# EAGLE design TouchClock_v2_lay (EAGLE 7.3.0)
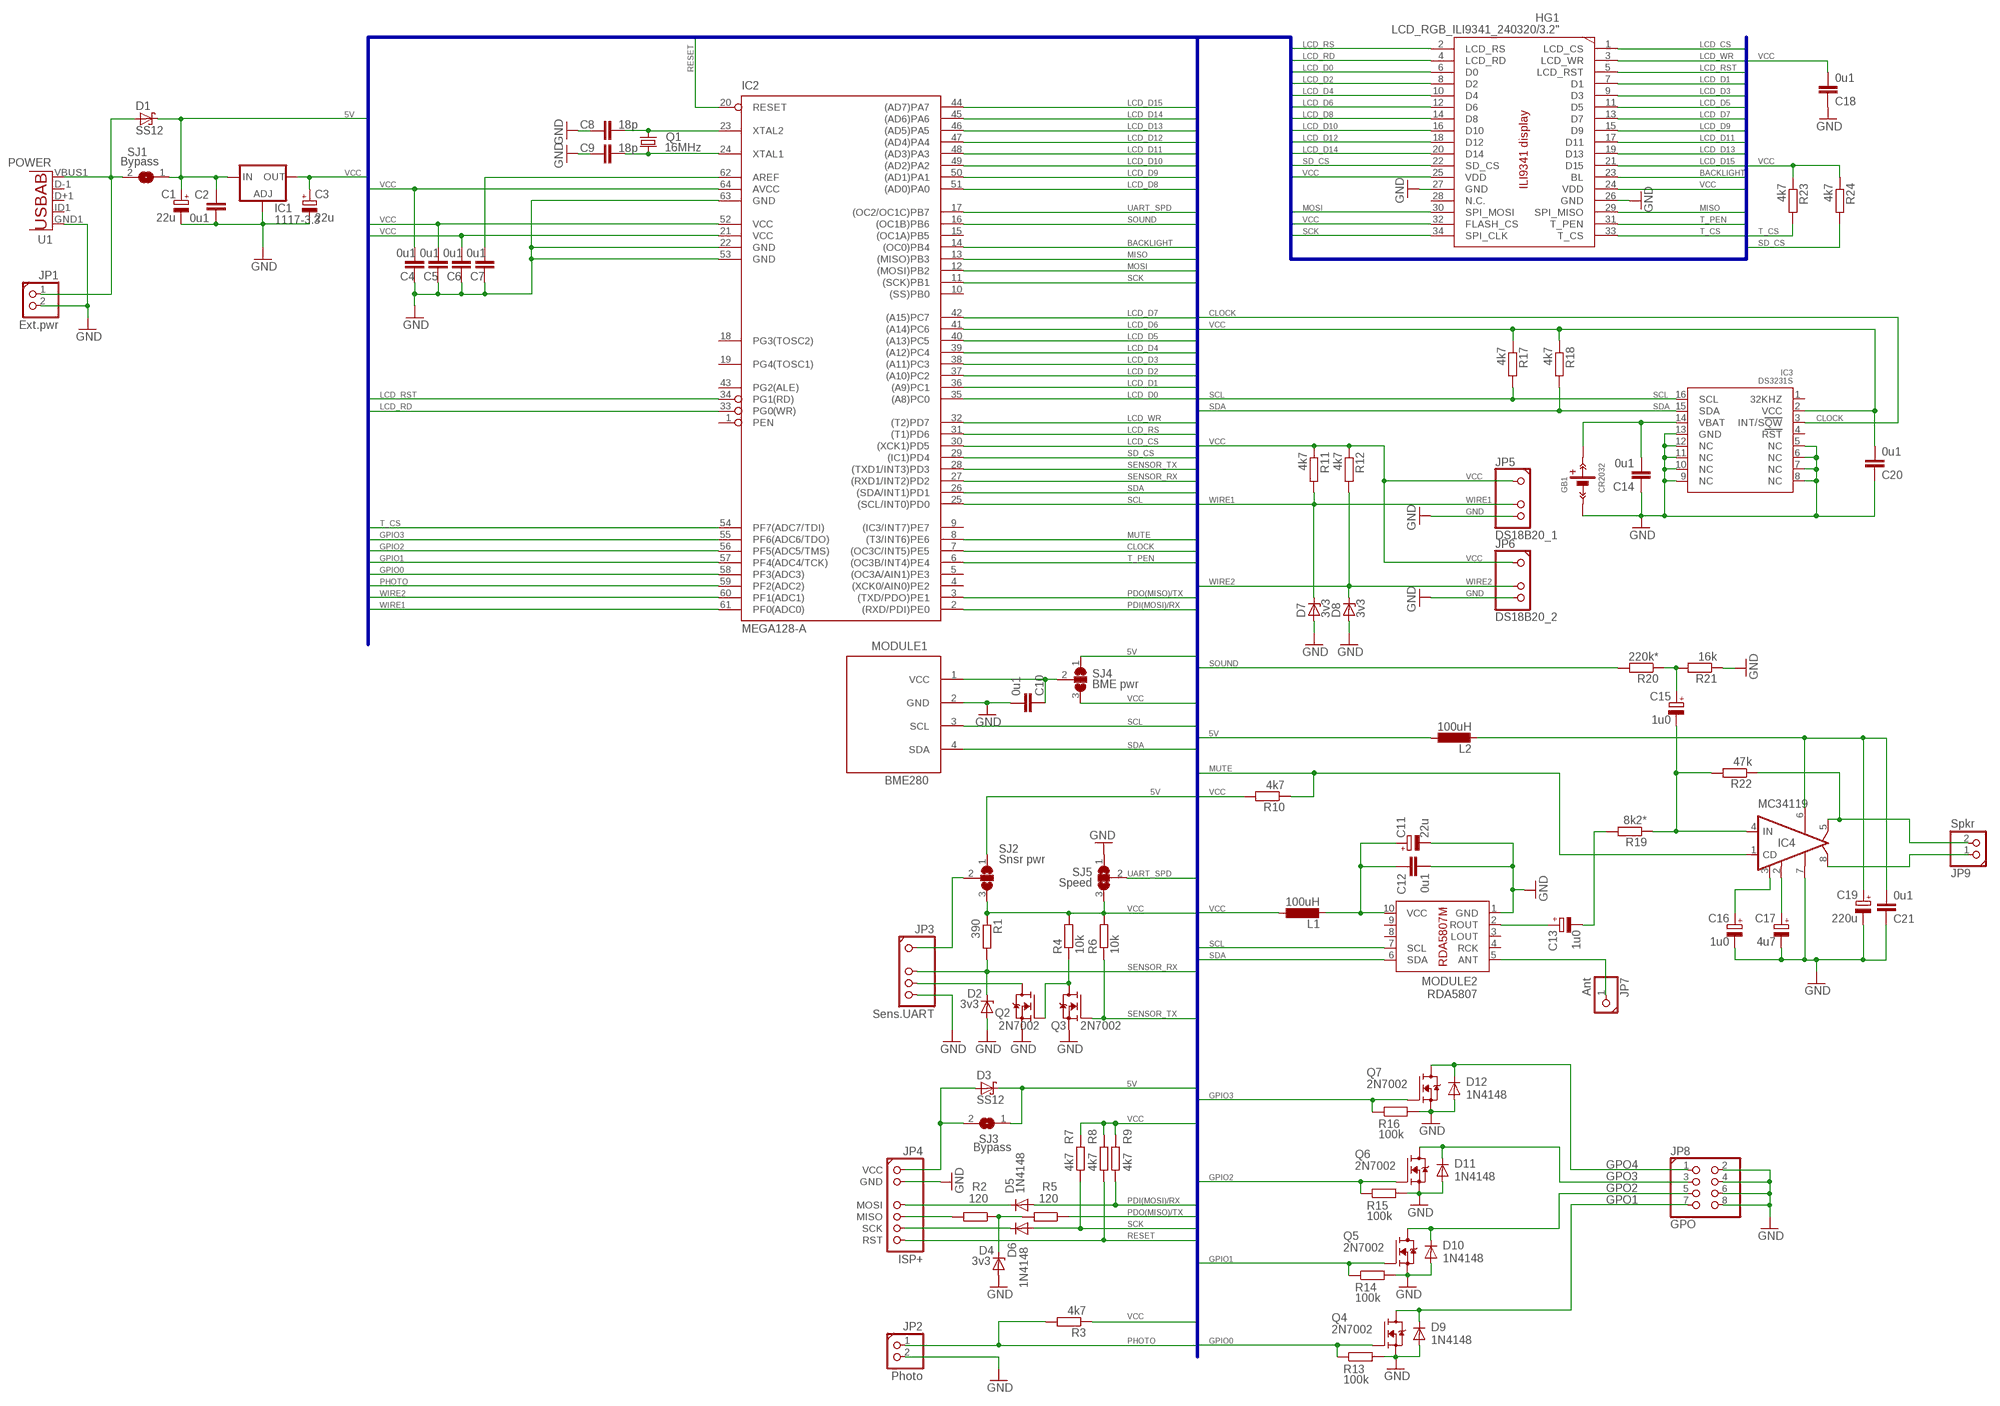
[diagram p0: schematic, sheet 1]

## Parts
C1  22u  CPOL-EUSMCB  [SMC_B]
C2  0u1  C-EUC0805T  [C0805T]
C3  22u  CPOL-EUSMCB  [SMC_B]
C4  0u1  C-EUC0805T  [C0805T]
C5  0u1  C-EUC0805T  [C0805T]
C6  0u1  C-EUC0805T  [C0805T]
C7  0u1  C-EUC0805T  [C0805T]
C8  18p  C-EUC0805T  [C0805T]
C9  18p  C-EUC0805T  [C0805T]
C10  0u1  C-EUC0805T  [C0805T]
C11  22u  CPOL-EUSMCB  [SMC_B]
C12  0u1  C-EUC0805T  [C0805T]
C13  1u0  CPOL-EUSMCB  [SMC_B]
C14  0u1  C-EUC0805T  [C0805T]
C15  1u0  CPOL-EUSMCB  [SMC_B]
C16  1u0  CPOL-EUSMCB  [SMC_B]
C17  4u7  CPOL-EUSMCB  [SMC_B]
C18  0u1  C-EUC0805T  [C0805T]
C19  220u  CPOL-EU153CLV-0605  [153CLV-0605]
C20  0u1  C-EUC0805T  [C0805T]
C21  0u1  C-EUC0805T  [C0805T]
D1  SS12  SS_XXX  [SMA(214AC)]
D2  3v3  ZENER-DIODESMB  [SMB(214AA)]
D3  SS12  SS_XXX  [SMA(214AC)]
D4  3v3  ZENER-DIODESOD80C  [SOD80C]
D5  1N4148  1N4148SMD  [SOD80-R]
D6  1N4148  1N4148SMD  [SOD80-R]
D7  3v3  ZENER-DIODESMB  [SMB(214AA)]
D8  3v3  ZENER-DIODESMB  [SMB(214AA)]
D9  1N4148  1N4148SMD  [SOD80-R]
D10  1N4148  1N4148SMD  [SOD80-R]
D11  1N4148  1N4148SMD  [SOD80-R]
D12  1N4148  1N4148SMD  [SOD80-R]
GB1  CR2032  CR2032_HOLDER/CH224  [CH224-2032]
HG1  LCD_RGB_ILI9341_240320/3.2"  [3"2_320*240_ILI9341]
IC1  1117-3.3  LD117AS33TR  [SOT223]
IC2  MEGA128-A  [TQFP64]
IC3  DS3231S  [SO16W]
IC4  MC34119  MC34119D  [SO08]
JP1  Ext.pwr  CONN1X2/R  [1X02ROUND]
JP2  Photo  CONN1X2/R  [1X02ROUND]
JP3  Sens.UART  CONN1X5(1+3)90R  [1X05ROUND/90(1+3)]
JP4  ISP+  CONN1X7(2+4)_ISP+/R90  [1X07/90/R_ISP+]
JP5  DS18B20_1  CONN1X4(1+2)/R90  [1X04ROUND/90(1+2)]
JP6  DS18B20_2  CONN1X4(1+2)/R90  [1X04ROUND/90(1+2)]
JP7  Ant  CONN1X1/R90  [1X01ROUND/90]
JP8  GPO  CONN2X4/R  [2X04ROUND]
JP9  Spkr  CONN1X2/R90  [1X02ROUND/90]
L1  100uH  L-EUL1812  [L1812]
L2  100uH  L-EUL1812  [L1812]
MODULE1  BME280  BM(P|E)280_I2C/4  [BM(P|E)280_I2C_5V]
MODULE2  RDA5807  RDA5807M/PAD  [RDA5807_MODULE_PADS]
Q1  16MHz  CRYSTALSM49  [SM49]
Q2  2N7002  2N7002/THIN  [SOT23_THIN]
Q3  2N7002  2N7002/THIN  [SOT23_THIN]
Q4  2N7002  2N7002/THIN  [SOT23_THIN]
Q5  2N7002  2N7002/THIN  [SOT23_THIN]
Q6  2N7002  2N7002/THIN  [SOT23_THIN]
Q7  2N7002  2N7002/THIN  [SOT23_THIN]
R1  390  R-EU_R0805T  [R0805T]
R2  120  R-EU_R0805T  [R0805T]
R3  4k7  R-EU_R0805T  [R0805T]
R4  10k  R-EU_R0805T  [R0805T]
R5  120  R-EU_R0805T  [R0805T]
R6  10k  R-EU_R0805T  [R0805T]
R7  4k7  R-EU_R0805T  [R0805T]
R8  4k7  R-EU_R0805T  [R0805T]
R9  4k7  R-EU_R0805T  [R0805T]
R10  4k7  R-EU_R0805T  [R0805T]
R11  4k7  R-EU_R0805T  [R0805T]
R12  4k7  R-EU_R0805T  [R0805T]
R13  100k  R-EU_R0805T  [R0805T]
R14  100k  R-EU_R0805T  [R0805T]
R15  100k  R-EU_R0805T  [R0805T]
R16  100k  R-EU_R0805T  [R0805T]
R17  4k7  R-EU_R0805T  [R0805T]
R18  4k7  R-EU_R0805T  [R0805T]
R19  8k2*  R-EU_R0805T  [R0805T]
R20  220k*  R-EU_R0805T  [R0805T]
R21  16k  R-EU_R0805T  [R0805T]
R22  47k  R-EU_R0805T  [R0805T]
R23  4k7  R-EU_R0805T  [R0805T]
R24  4k7  R-EU_R0805T  [R0805T]
SJ1  Bypass  SJ/NS  [SJ_NOSILK]
SJ2  Snsr pwr  SJ2W  [SJ_2]
SJ3  Bypass  SJ/NS  [SJ_NOSILK]
SJ4  BME pwr  SJ2W  [SJ_2]
SJ5  Speed  SJ2W  [SJ_2]
U1  POWER  USB5""  [USB-MICRO-SMD]

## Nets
5V: C1.+ C2.1 D1.C D3.C IC1.3(IN) L2.1 SJ1.1 SJ2.1 SJ3.1 SJ4.1
BACKLIGHT: HG1.23(BL) IC2.14((OC0)PB4)
CLOCK: IC2.7((OC3C/INT5)PE5) IC3.3(INT/SQW)
GND: C1.- C2.2 C3.- C4.1 C5.1 C6.1 C7.1 C8.1 C9.1 C10.2 C11.- C12.2 C14.1 C16.- C17.- C18.1 C19.- C20.1 C21.1 D2.A D4.A D7.A D8.A D9.A D10.A D11.A D12.A GB1.GB- HG1.26(GND) HG1.27(GND) IC1.1(ADJ) IC2.22(GND) IC2.53(GND) IC2.63(GND) IC3.5(NC) IC3.6(NC) IC3.7(NC) IC3.8(NC) IC3.9(NC) IC3.10(NC) IC3.11(NC) IC3.12(NC) IC3.13(GND) IC4.7(GND) JP1.2 JP2.2 JP3.5 JP4.GND JP5.4 JP6.4 JP8.2 JP8.4 JP8.6 JP8.8 MODULE1.2(GND) MODULE2.1(GND) Q2.2(S) Q3.2(S) Q4.2(S) Q5.2(S) Q6.2(S) Q7.2(S) R13.2 R14.2 R15.2 R16.2 R21.1 SJ5.1 U1.GND1(GND)
GPIO0: IC2.58(PF3(ADC3)) Q4.1(G) R13.1
GPIO1: IC2.57(PF4(ADC4/TCK)) Q5.1(G) R14.1
GPIO2: IC2.56(PF5(ADC5/TMS)) Q6.1(G) R15.1
GPIO3: IC2.55(PF6(ADC6/TDO)) Q7.1(G) R16.1
GPO1: D9.C JP8.7 Q4.3(D)
GPO2: D10.C JP8.5 Q5.3(D)
GPO3: D11.C JP8.3 Q6.3(D)
GPO4: D12.C JP8.1 Q7.3(D)
LCD_CS: HG1.1(LCD_CS) IC2.30((XCK1)PD5)
LCD_D0: HG1.6(D0) IC2.35((A8)PC0)
LCD_D1: HG1.7(D1) IC2.36((A9)PC1)
LCD_D2: HG1.8(D2) IC2.37((A10)PC2)
LCD_D3: HG1.9(D3) IC2.38((A11)PC3)
LCD_D4: HG1.10(D4) IC2.39((A12)PC4)
LCD_D5: HG1.11(D5) IC2.40((A13)PC5)
LCD_D6: HG1.12(D6) IC2.41((A14)PC6)
LCD_D7: HG1.13(D7) IC2.42((A15)PC7)
LCD_D8: HG1.14(D8) IC2.51((AD0)PA0)
LCD_D9: HG1.15(D9) IC2.50((AD1)PA1)
LCD_D10: HG1.16(D10) IC2.49((AD2)PA2)
LCD_D11: HG1.17(D11) IC2.48((AD3)PA3)
LCD_D12: HG1.18(D12) IC2.47((AD4)PA4)
LCD_D13: HG1.19(D13) IC2.46((AD5)PA5)
LCD_D14: HG1.20(D14) IC2.45((AD6)PA6)
LCD_D15: HG1.21(D15) IC2.44((AD7)PA7)
LCD_RD: HG1.4(LCD_RD) IC2.33(PG0(WR))
LCD_RS: HG1.2(LCD_RS) IC2.31((T1)PD6)
LCD_RST: HG1.5(LCD_RST) IC2.34(PG1(RD))
LCD_WR: HG1.3(LCD_WR) IC2.32((T2)PD7)
MISO: HG1.29(SPI_MISO) IC2.13((MISO)PB3)
MOSI: HG1.30(SPI_MOSI) IC2.12((MOSI)PB2)
MUTE: IC2.8((T3/INT6)PE6) IC4.1(CD) R10.1
N$1: C9.2 IC2.24(XTAL1) Q1.2
N$2: C8.2 IC2.23(XTAL2) Q1.1
N$3: C7.2 IC2.62(AREF)
N$4: JP4.MISO R2.2
N$5: C16.+ IC4.3(FC1)
N$6: C11.+ C12.1 L1.2 MODULE2.10(VCC)
N$7: C17.+ IC4.2(FC2)
N$8: JP7.1 MODULE2.5(ANT)
N$9: C13.+ MODULE2.2(ROUT)
N$10: C13.- R19.2
N$11: C19.+ C21.2 IC4.6(VCC) L2.2
N$12: C15.+ R20.1 R21.2
N$13: C15.- IC4.4(IN) R19.1 R22.2
N$14: IC4.8(VO2) JP9.1
N$15: IC4.5(VO1) JP9.2 R22.1
N$16: JP3.1 SJ2.2
N$17: JP3.4 Q2.3(D)
N$18: D4.C R2.1 R5.2
N$19: Q2.1(G) Q3.3(D) R4.1
N$20: C10.1 MODULE1.1(VCC) SJ4.2
N$23: D3.A JP4.+5V(VCC) SJ3.2
N$25: D5.C JP4.MOSI
N$26: D6.C JP4.SCK
PDI(MOSI)/RX: D5.A IC2.2((RXD/PDI)PE0) R9.2
PDO(MISO)/TX: IC2.3((TXD/PDO)PE1) R5.1
PHOTO: IC2.59(PF2(ADC2)) JP2.1 R3.2
RESET: IC2.20(RESET) JP4.RST R8.2
SCK: D6.A HG1.34(SPI_CLK) IC2.11((SCK)PB1) R7.2
SCL: IC2.25((SCL/INT0)PD0) IC3.16(SCL) MODULE1.3(SCL) MODULE2.7(SCL) R17.2
SD_CS: HG1.22(SD_CS) IC2.29((IC1)PD4) R24.2
SDA: IC2.26((SDA/INT1)PD1) IC3.15(SDA) MODULE1.4(SDA) MODULE2.6(SDA) R18.2
SENSOR_RX: D2.C IC2.27((RXD1/INT2)PD2) JP3.3 R1.2
SENSOR_TX: IC2.28((TXD1/INT3)PD3) Q3.1(G) R6.1
SOUND: IC2.16((OC1B)PB6) R20.2
SUPPLY: D1.A JP1.1 SJ1.2 U1.VBUS1(VBUS)
T_CS: HG1.33(T_CS) IC2.54(PF7(ADC7/TDI)) R23.2
T_PEN: HG1.31(T_PEN) IC2.6((OC3B/INT4)PE4)
UART_SPD: IC2.17((OC2/OC1C)PB7) SJ5.2
VBAT: C14.2 GB1.GB+ IC3.14(VBAT)
VCC: C3.+ C4.2 C5.2 C6.2 C18.2 C20.2 HG1.24(VDD) HG1.25(VDD) HG1.32(FLASH_CS) IC1.4(OUT) IC2.21(VCC) IC2.52(VCC) IC2.64(AVCC) IC3.2(VCC) JP5.1 JP6.1 L1.1 R1.1 R3.1 R4.2 R6.2 R7.1 R8.1 R9.1 R10.2 R11.1 R12.1 R17.1 R18.1 R23.1 R24.1 SJ2.3 SJ4.3 SJ5.3
WIRE1: D7.C IC2.61(PF0(ADC0)) JP5.3 R11.2
WIRE2: D8.C IC2.60(PF1(ADC1)) JP6.3 R12.2
Unconnected: HG1.28(N.C.) IC2.1(PEN) IC2.4((XCK0/AIN0)PE2) IC2.5((OC3A/AIN1)PE3) IC2.9((IC3/INT7)PE7) IC2.10((SS)PB0) IC2.15((OC1A)PB5) IC2.18(PG3(TOSC2)) IC2.19(PG4(TOSC1)) IC2.43(PG2(ALE)) IC3.1(32KHZ) IC3.4(RST) MODULE2.3(LOUT) MODULE2.4(RCK) MODULE2.8(NC1) MODULE2.9(NC2) U1.D+1(D+) U1.D-1(D-) U1.ID1(USBID)

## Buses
5V,VCC,LCD_CS,LCD_WR,LCD_RD,LCD_RST,LCD_RS,LCD_D[0..15],MISO,MOSI,SCK,PDI(MOSI)/RX,PDO(MISO)/TX,T_PEN,T_CS,SD_CS,BACKLIGHT,RESET,SCL,SDA,WIRE1,WIRE2,CLOCK,SOUND,MUTE,SENSOR_RX,SENSOR_TX,GPIO[0..3],PHOTO,UART_SPD

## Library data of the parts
C1 C3 C11 C13 C15-C17 C19 = rcl:CPOL-EU: POLARIZED CAPACITOR, European symbol
C2 C4-C10 C12 C14 C18 C20 C21 = rcl:C-EU: CAPACITOR, European symbol
D1 D3 = diode:SS_XXX: SS12 -13 -14 -15 -16 -18 -19 -100
D2 D4 D7 D8 = diode:ZENER-DIODE: Z-Diode
D5 D6 D9-D12 = diode:1N4148: DIODE
GB1 = misc_passive_AL:CR2032_HOLDER: CR2032 Holder
HG1 = lcd-AL:LCD_RGB_ILI9341_240*320
IC1 = v-reg:LD117A?*: Low drop fixed and adjustable positive voltage regulators 1 A Source: http://www.st.com/stonline/products/literature/ds/7194/ld1117axx.pdf
IC2 = atmel:MEGA128: MICROCONTROLLER 128 Kbytes FLASH 4 Kbytes SRAM 4 Kbytes EEPROM DUAL USART 8-channel 10 bit ADC Source: avr.lbr; MPN: ATMEGA128-16AU; OC_FARNELL: 9171118; OC_NEWARK: 95K7364
IC3 = misc-active-AL:DS3231S: TCXO Clock
IC4 = misc-active-AL:MC34119: Low Power Audio Amplifier Motorola
JP1 JP2 JP9 = pinhead-AL:CONN1X2: PIN HEADER
JP3 = pinhead-AL:CONN1X5(1+3)
JP4 = pinhead-AL:CONN1X7(2+4)_ISP+: PIN HEADER
JP5 JP6 = pinhead-AL:CONN1X4(1+2)
JP7 = pinhead-AL:CONN1X1
JP8 = pinhead-AL:CONN2X4: PIN HEADER
L1 L2 = rcl:L-EU: INDUCTOR, European symbol
MODULE1 = modules-external-AL:BM(P|E)280_I2C
MODULE2 = modules-external-AL:RDA5807M
Q1 = crystal:CRYSTAL: CRYSTAL; OC_FARNELL: unknown; OC_NEWARK: unknown
Q2-Q7 = transistor-fet:2N7002: Small signal N-Channel MOSFET transistor
R1-R24 = rcl:R-EU_: RESISTOR, European symbol
SJ1 SJ3 = jumper:SJ: SMD solder JUMPER
SJ2 SJ4 SJ5 = jumper:SJ2W: SMD solder JUMPER
U1 = usb:USB5: This is a USB AB connector that is compatible with USB OTG. i.e. this connector can serve as a host or device

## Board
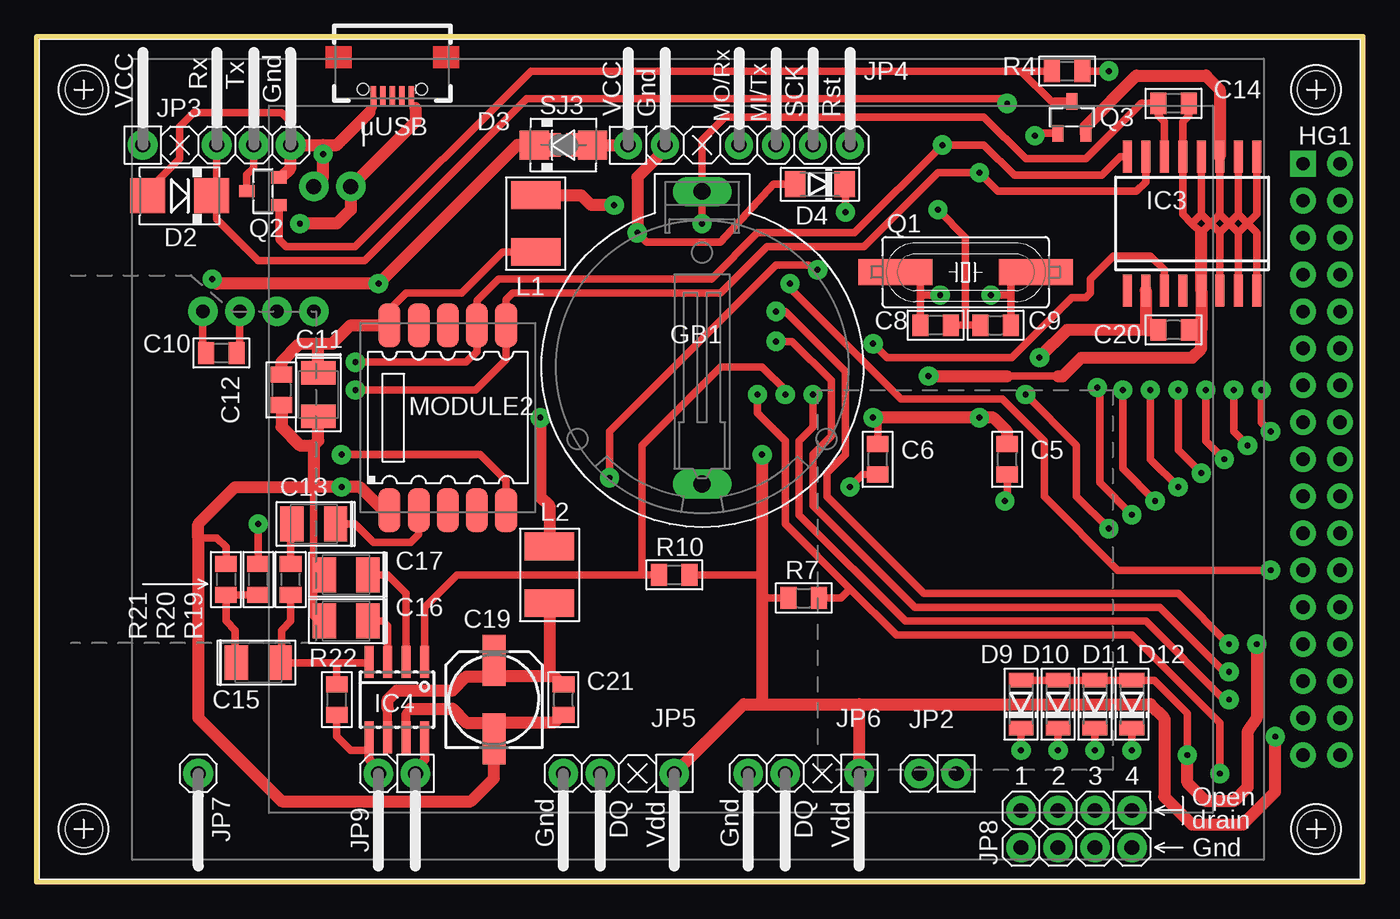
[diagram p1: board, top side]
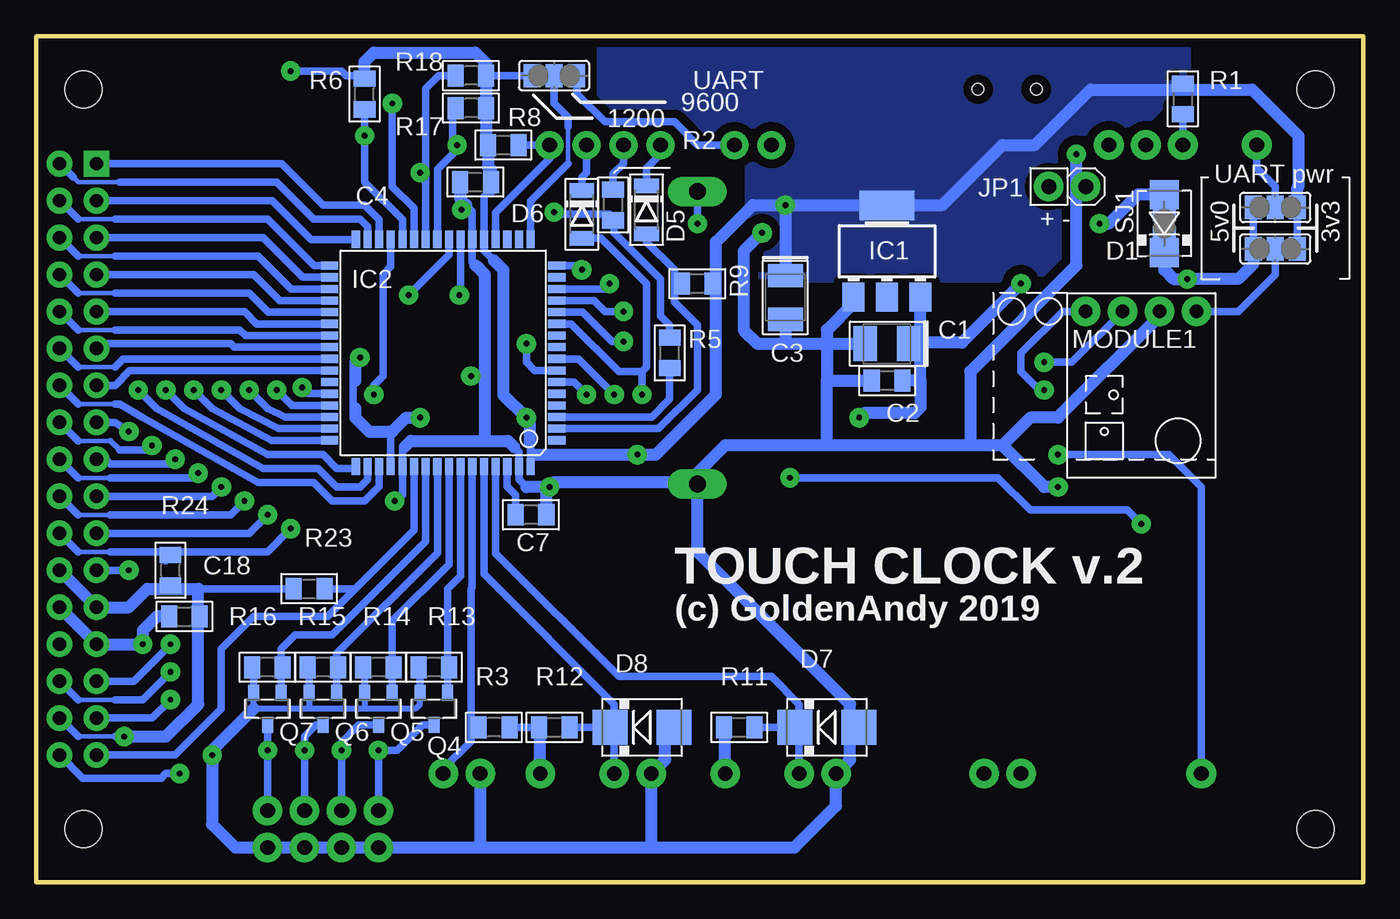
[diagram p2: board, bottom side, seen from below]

Size 91.12 x 58.1 mm. Coordinates in mm from the lower left corner, seen from the top.
Outline: 0,58.1 91.12,58.1 91.12,0 0,0 0,58.1
Copper layers (1*16): Top 0.035mm / dielectric 1.5mm / Bottom 0.035mm
Design rules "default *": minimum track width 12mil, minimum drill 14mil, track to track 8mil, track to pad 8mil, pad to pad 8mil, via to via 8mil, smd to smd 8mil, copper to edge 20mil, drill to drill 30mil, minimum pad ring 16mil, minimum via ring 18mil, stop-mask expansion 4mil, vias tented up to drill 0mil, thermal gap 16mil
Holes 2.54 mm at 3.25,54.45 87.89,54.45 87.89,3.65 3.25,3.65

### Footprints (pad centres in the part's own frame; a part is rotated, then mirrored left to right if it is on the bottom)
SMC_B = smd 1.6 x 2.4: + -1.5,0; - 1.5,0
C0805T = smd 1.1 x 1.5: 1 -1.05,0; 2 1.05,0
153CLV-0605 = smd 3.5 x 1.6: + 2.7,0; - -2.7,0
SMA(214AC) = smd 2 x 2: A 2,0; C -2,0
SMB(214AA) = smd 2.4 x 2.4: A 2.2,0; C -2.2,0
SOD80C = smd 1.4 x 1.8: A 1.7,0; C -1.7,0
SOD80-R = smd 1 x 1.7: A 1.65,0; C -1.65,0
CH224-2032 = drill 1.143 pad 2.032 long: GB+ -12.05,0; GB- 8.05,0
3"2_320*240_ILI9341 = drill 0.9 pad 1.778 square: 1 32.703,20.32 | drill 0.9 pad 1.778: 2 35.242,20.32; 3 32.703,17.78; 4 35.242,17.78; 5 32.703,15.24; 6 35.242,15.24; 7 32.703,12.7; 8 35.242,12.7; 9 32.703,10.16; 10 35.242,10.16; 11 32.703,7.62; 12 35.242,7.62; 13 32.703,5.08; 14 35.242,5.08; 15 32.703,2.54; 16 35.242,2.54; 17 32.703,0; 18 35.242,0; 19 32.703,-2.54; 20 35.242,-2.54; 21 32.703,-5.08; 22 35.242,-5.08; 23 32.703,-7.62; 24 35.242,-7.62; 25 32.703,-10.16; 26 35.242,-10.16; 27 32.703,-12.7; 28 35.242,-12.7; 29 32.703,-15.24; 30 35.242,-15.24; 31 32.703,-17.78; 32 35.242,-17.78; 33 32.703,-20.32; 34 35.242,-20.32
SOT223 = smd 1.5 x 2: 1 -2.3,-3.15; 2 0,-3.15; 3 2.3,-3.15 | smd 3.8 x 2: 4 0,3.15
TQFP64 = smd 1.194 x 0.559: 1 -7.8,6; 2 -7.8,5.2; 3 -7.8,4.4; 4 -7.8,3.6; 5 -7.8,2.8; 6 -7.8,2; 7 -7.8,1.2; 8 -7.8,0.4; 9 -7.8,-0.4; 10 -7.8,-1.2; 11 -7.8,-2; 12 -7.8,-2.8; 13 -7.8,-3.6; 14 -7.8,-4.4; 15 -7.8,-5.2; 16 -7.8,-6; 33 7.8,-6; 34 7.8,-5.2; 35 7.8,-4.4; 36 7.8,-3.6; 37 7.8,-2.8; 38 7.8,-2; 39 7.8,-1.2; 40 7.8,-0.4; 41 7.8,0.4; 42 7.8,1.2; 43 7.8,2; 44 7.8,2.8; 45 7.8,3.6; 46 7.8,4.4; 47 7.8,5.2; 48 7.8,6 | smd 0.559 x 1.194: 17 -6,-7.8; 18 -5.2,-7.8; 19 -4.4,-7.8; 20 -3.6,-7.8; 21 -2.8,-7.8; 22 -2,-7.8; 23 -1.2,-7.8; 24 -0.4,-7.8; 25 0.4,-7.8; 26 1.2,-7.8; 27 2,-7.8; 28 2.8,-7.8; 29 3.6,-7.8; 30 4.4,-7.8; 31 5.2,-7.8; 32 6,-7.8; 49 6,7.8; 50 5.2,7.8; 51 4.4,7.8; 52 3.6,7.8; 53 2.8,7.8; 54 2,7.8; 55 1.2,7.8; 56 0.4,7.8; 57 -0.4,7.8; 58 -1.2,7.8; 59 -2,7.8; 60 -2.8,7.8; 61 -3.6,7.8; 62 -4.4,7.8; 63 -5.2,7.8; 64 -6,7.8
SO16W = smd 0.6 x 2.2: 1 -4.445,-4.6; 2 -3.175,-4.6; 3 -1.905,-4.6; 4 -0.635,-4.6; 5 0.635,-4.6; 6 1.905,-4.6; 7 3.175,-4.6; 8 4.445,-4.6; 9 4.445,4.6; 10 3.175,4.6; 11 1.905,4.6; 12 0.635,4.6; 13 -0.635,4.6; 14 -1.905,4.6; 15 -3.175,4.6; 16 -4.445,4.6
SO08 = smd 0.6 x 2.2: 1 -1.905,-2.6; 2 -0.635,-2.6; 3 0.635,-2.6; 4 1.905,-2.6; 5 1.905,2.6; 6 0.635,2.6; 7 -0.635,2.6; 8 -1.905,2.6
1X02ROUND = drill 1.016 pad 2.032: 1 -1.27,0; 2 1.27,0
1X05ROUND/90(1+3) = drill 1.016 pad 2.032: 1 -5.08,0; 3 0,0; 4 2.54,0; 5 5.08,0
1X07/90/R_ISP+ = drill 1.016 pad 1.93: +5V -7.62,0; GND -5.08,0; MISO 2.54,0; MOSI 0,0; RST 7.62,0; SCK 5.08,0
1X04ROUND/90(1+2) = drill 1.016 pad 2.032: 1 -3.81,0; 3 1.27,0; 4 3.81,0
1X01ROUND/90 = drill 1.016 pad 2.032: 1 0,0
2X04ROUND = drill 1.016 pad 2.032: 1 -3.81,-1.27; 2 -3.81,1.27; 3 -1.27,-1.27; 4 -1.27,1.27; 5 1.27,-1.27; 6 1.27,1.27; 7 3.81,-1.27; 8 3.81,1.27
1X02ROUND/90 = drill 1.016 pad 2.032: 1 -1.27,0; 2 1.27,0
L1812 = smd 1.9 x 3.4: 1 -1.95,0; 2 1.95,0
BM(P|E)280_I2C_5V = drill 0.914 pad 2.032: 1 3.81,5.08; 2 1.27,5.08; 3 -1.27,5.08; 4 -3.81,5.08
RDA5807_MODULE_PADS = smd 3.048 x 1.524: 1 -6.35,4; 2 -6.35,2; 3 -6.35,0; 4 -6.35,-2; 5 -6.35,-4; 6 6.35,-4; 7 6.35,-2; 8 6.35,0; 9 6.35,2; 10 6.35,4
SM49 = smd 5.08 x 1.778: 1 -4.826,0; 2 4.826,0
SOT23_THIN = smd 0.8 x 1.1: 1 -0.95,-1.1; 2 0.95,-1.1; 3 0,1.1
R0805T = smd 1.1 x 1.5: 1 -1.05,0; 2 1.05,0
SJ_NOSILK = smd 1.168 x 1.6: 1 -0.762,0; 2 0.762,0
SJ_2 = smd 1.168 x 1.6: 1 -1.524,0; 2 0,0; 3 1.524,0
USB-MICRO-SMD = smd 1.4 x 0.4: D+1 2.7,0; D-1 2.7,0.65; GND1 2.7,-1.3; ID1 2.7,-0.65; VBUS1 2.7,1.3 | hole 0.8: 2.2,2; 2.2,-2

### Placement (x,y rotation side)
C1  32.7,36.99 180 bottom
C2  32.7,34.45 180 bottom
C3  39.69,40.16 270 bottom
C4  60.96,48.1 0 bottom
C5  66.67,29.05 90 top
C6  57.79,29.05 90 top
C7  57.15,25.24 180 bottom
C8  61.75,38.26 180 top
C9  65.88,38.26 0 top
C10  12.7,36.35 0 top
C11  19.37,33.5 270 top
C12  16.83,33.81 270 top
C13  19.05,24.61 180 top
C14  78.11,53.5 180 top
C15  15.24,15.08 0 top
C16  21.27,17.94 180 top
C17  21.27,21.11 180 top
C18  80.96,18.26 0 bottom
C19  31.43,12.54 90 top
C20  78.11,37.94 180 top
C21  36.2,12.54 90 top
D1  13.65,45.24 90 bottom
D2  9.84,47.15 180 top
D3  36.2,50.64 0 top
D4  53.82,47.94 180 top
D5  49.21,46.2 270 bottom
D6  53.66,45.88 270 bottom
D7  36.83,10.64 0 bottom
D8  49.53,10.64 0 bottom
D9  67.63,12.22 90 top
D10  70.17,12.22 90 top
D11  72.71,12.22 90 top
D12  75.25,12.22 90 top
GB1  45.72,35.4 270 top
HG1  54.29,29.05 0 top
IC1  32.7,43.34 0 bottom
IC2  63.18,36.35 180 bottom
IC3  79.38,45.24 0 top
IC4  24.77,12.54 180 top
JP1  20.32,47.78 0 bottom
JP2  61.91,7.46 180 top
JP3  12.38,50.64 0 top
JP4  48.26,50.64 0 top
JP5  40.01,7.46 180 top
JP6  52.71,7.46 180 top
JP7  11.11,7.46 180 top
JP8  71.44,3.65 180 top
JP9  24.77,7.46 180 top
L1  34.29,45.24 270 top
L2  35.24,21.11 270 top
MODULE1  15.24,34.13 0 bottom
MODULE2  28.26,31.91 90 top
Q1  63.82,41.91 0 top
Q2  15.56,47.47 90 top
Q3  71.12,52.55 0 top
Q4  63.82,11.91 180 bottom
Q5  67.63,11.91 180 bottom
Q6  71.44,11.91 180 bottom
Q7  75.25,11.91 180 bottom
R1  12.38,53.82 270 bottom
R2  51.51,46.51 90 bottom
R3  59.69,10.64 180 bottom
R4  70.8,55.72 0 top
R5  47.62,36.35 90 bottom
R6  68.58,54.13 90 bottom
R7  52.71,19.53 0 top
R8  59.05,50.64 0 bottom
R9  45.72,41.12 180 bottom
R10  43.82,21.11 0 top
R11  42.86,10.64 0 bottom
R12  55.56,10.64 0 bottom
R13  63.82,14.76 180 bottom
R14  67.63,14.76 180 bottom
R15  71.44,14.76 180 bottom
R16  75.25,14.76 180 bottom
R17  61.28,53.18 180 bottom
R18  61.28,55.4 180 bottom
R19  17.46,20.8 90 top
R20  15.24,20.8 90 top
R21  13.02,20.8 270 top
R22  20.64,12.54 90 top
R23  72.39,20.16 0 bottom
R24  81.92,21.43 90 bottom
SJ1  13.65,45.24 90 bottom
SJ2  6.03,46.36 0 bottom
SJ3  36.2,50.64 0 top
SJ4  6.03,43.5 0 bottom
SJ5  55.56,55.4 180 bottom
U1  24.45,56.67 270 top

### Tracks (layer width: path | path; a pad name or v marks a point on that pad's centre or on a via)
5V  (via drill 0.41)
  Top 0.813: v34.61,31.91 34.61,26.51 35.24,25.88 L2.1 | SJ3.1 D3.C 33.02,50.64 v23.5,41.12 12.38,41.12 v12.07,41.43
  Bottom 0.508: SJ4.1 SJ2.1
  Bottom 0.813: 30.4,34.45 30.8,34.45 C2.1 | 30.4,34.45 30.4,32.62 30.8,32.23 34.29,32.23 v34.61,31.91 | v23.5,41.12 27.54,37.07 30.16,37.07 30.4,37.31 | 30.4,34.45 30.4,36.99 | 30.4,36.99 30.4,37.31 | 30.4,37.31 IC1.3 | C1.+ 30.4,36.99 | SJ4.1 7.56,42.45 8.57,41.43 v12.07,41.43 13.02,41.43 13.65,42.07 D1.C SJ1.1
BACKLIGHT  (via drill 0.41)
  Top 0.508: v84.77,21.43 74.3,21.43 69.22,26.51 69.22,30.32 66.36,33.18 59.37,33.18 51.75,40.8 v51.75,41.12
  Bottom 0.508: HG1.23 v84.77,21.43 | IC2.14 52.12,40.75 v51.75,41.12
CLOCK  (via drill 0.41)
  Top 0.508: v57.47,36.99 58.42,36.04 66.99,36.04 71.12,40.16 72.07,40.16 72.39,40.48 72.39,41.43 73.98,43.02 76.52,43.02 77.47,42.07 IC3.3
  Bottom 0.508: IC2.7 56.9,35.15 57.47,35.72 v57.47,36.99
GND  (via drill 0.41)
  Top 0.406: U1.GND1 23.15,53.15 22.86,52.86
  Top 0.508: C9.1 63.82,38.26 | 63.82,38.26 C8.1 | C6.1 56.73,28 v55.88,27.15 | C5.1 66.67,26.67 v66.52,26.19 | IC3.8 83.82,44.61 82.55,45.88 | 82.55,45.88 IC3.10 | IC3.7 82.55,44.61 | 82.55,44.61 81.28,45.88 | 81.28,45.88 IC3.11 | IC3.6 81.28,44.61 | 81.28,44.61 80.01,45.88 | 80.01,45.88 IC3.12 | 79.38,45.24 80.01,44.61 81.28,45.88 | 79.38,45.24 78.74,45.88 IC3.13 78.74,52.23 79.16,52.64 C14.1 | 80.01,45.88 79.38,45.24 | 81.28,44.61 82.55,45.88 | 82.55,44.61 83.82,45.88 IC3.9 | 66.67,34.77 70.17,34.77 | 63.82,38.26 63.82,44.29 v61.91,46.2 | Q2.2 16.82,48.42 | D9.A D10.A D11.A D12.A 76.77,13.87 79.06,11.59 v79.06,8.73 | C16.- 19.37,17.94 19.05,18.26 19.05,21.11 | 19.05,21.11 19.05,27.15 | C17.- 19.05,21.11 | R21.1 13.02,23.02 12.38,23.65 11.11,23.65 | MODULE1.2 13.97,36.57 C10.2 | JP3.5 17.46,52.23 16.83,52.86 10.8,52.86 9.84,51.91 9.84,49.69 7.64,47.49 D2.A | D4.A 50.64,47.94 46.99,43.97 41.91,43.97 v41.28,44.61
  Top 0.61: IC4.7 25.4,11.59 25.72,11.91
  Top 0.813: 80.01,44.61 IC3.5 80.01,37.94 | 80.01,37.94 C20.1 | v61.28,34.77 66.67,34.77 | 70.17,34.77 70.48,34.77 71.76,36.04 79.38,36.04 80.01,36.67 80.01,37.94 | 22.86,52.86 20.64,50.64 19.68,50.64 | MODULE2.1 23.81,25.56 22.22,27.15 v20.95,27.15 19.05,27.15 | C11.- 19.37,30.32 19.05,30 | C12.2 16.83,31.27 18.1,30 19.05,30 | 19.68,50.64 JP3.5 17.46,49.05 16.82,48.42 | IC3.11 81.28,54.45 80.33,55.4 75.56,55.4 72.07,51.91 Q3.2 | v83.82,16.35 83.82,11.27 83.19,10.32 83.19,6.51 82.23,5.56 80.33,5.56 79.06,6.83 v79.06,8.73 | JP4.GND 43.18,50.32 41.28,48.42 v41.28,44.61 | 25.72,11.91 28.57,11.91 29.53,10.95 31.11,10.95 | 31.11,10.95 31.11,10.16 C19.- 31.43,7.14 29.85,5.56 16.83,5.56 11.11,11.27 11.11,23.65 11.11,24.61 13.65,27.15 19.05,27.15 | C21.1 36.1,11.49 35.56,10.95 31.11,10.95 | 19.05,30 19.05,27.15 | JP1.2 19.68,48.42 v19.68,50.01 19.68,50.64
  Bottom 0.406: 68.58,11.91 65.09,11.91 64.77,12.22 Q4.2 | 68.58,11.91 72.39,11.91 | 72.39,11.91 76.2,11.91 Q7.2 | Q5.2 68.58,11.91 | Q6.2 72.39,11.91
  Bottom 0.508: 57.47,27.15 57.98,27.66 IC2.63 57.98,29.57 58.28,29.87 | 65.82,29.9 65.98,29.74 IC2.53 65.98,26.61 v66.52,26.19 | 60.96,42.39 61.18,42.61 IC2.22 61.18,46.1 61.59,46.51 v61.91,46.2 | v55.88,27.15 56.2,27.15 56.1,27.05 | Q4.2 64.77,14.66 R13.2 | Q5.2 68.58,14.66 R14.2 | Q6.2 72.39,14.66 R15.2 | Q7.2 76.2,14.66 R16.2 | 35.24,10.52 D7.A | GB1.GB- 45.83,27.35 | SJ5.1 53.98,55.4 53.98,54.13 52.07,52.23 47.31,52.23 45.72,50.64 JP4.GND
  Bottom 0.813: HG1.26 HG1.27 v83.82,16.35 83.82,17.3 82.87,18.26 C18.1 | 65.82,29.9 65.41,30.32 60.33,30.32 | 60.96,42.39 60.33,41.75 60.33,34.77 | 60.33,34.77 60.33,30.32 | 60.33,30.32 58.74,30.32 58.28,29.87 | 61.59,46.51 62.01,46.93 C4.1 | 56.2,27.15 57.47,27.15 | C7.1 56.1,27.05 | IC1.1 35,39.77 36.83,37.94 36.83,36.99 | 36.83,36.99 36.83,34.45 | 36.83,34.45 C2.2 | C3.- 39.69,36.99 | 39.69,36.99 36.83,36.99 | 36.83,36.99 C1.- | 26.99,30 26.99,35.08 19.68,42.39 v19.68,50.01 | 26.99,30 36.83,30 | 36.83,30 36.83,34.45 | v61.28,34.77 60.33,34.77 | 76.2,11.91 79.06,9.05 v79.06,8.73 79.06,3.97 77.47,2.38 JP8.2 JP8.4 JP8.6 JP8.8 60.64,2.38 | 36.83,30 43.82,30 45.72,28.1 GB1.GB- 45.72,22.7 35.24,12.22 35.24,10.52 35.24,8.41 JP5.4 36.2,5.24 39.05,2.38 48.9,2.38 | JP2.2 60.64,2.38 | 60.64,2.38 48.9,2.38 | 48.9,2.38 JP6.4 47.94,8.41 47.94,10.02 D8.A | 45.83,27.35 46.04,27.46 55.56,27.46 v55.88,27.15 | v41.28,44.61 42.55,43.34 42.55,37.94 41.59,36.99 39.69,36.99 | v20.95,27.15 21.91,27.15 24.77,30 | 24.77,30 26.99,30 | MODULE1.2 13.97,38.89 20.95,31.91 22.86,31.91 24.77,30
GPIO0
  Bottom 0.508: Q4.1 62.87,14.76 | 62.87,14.76 62.87,16.03 62.87,20.16 61.98,21.04 IC2.58 | R13.1 62.87,14.76
GPIO1
  Bottom 0.508: Q5.1 66.68,15.08 | 66.68,15.08 66.68,17.94 62.78,21.83 IC2.57 | R14.1 66.58,14.98 66.68,15.08
GPIO2
  Bottom 0.508: Q6.1 70.49,14.76 | 70.49,14.76 70.49,15.71 63.58,22.62 IC2.56 | R15.1 70.49,14.76
GPIO3
  Bottom 0.508: Q7.1 74.3,14.76 | 74.3,14.76 74.3,16.03 73.34,16.99 70.8,16.99 64.38,23.41 IC2.55 | R16.1 74.3,14.76
GPO1  (via drill 0.41)
  Top 0.508: D9.C v67.63,9.05
  Bottom 0.508: JP8.7 v67.63,9.05 66.36,9.05 64.6,10.81 Q4.3
GPO2  (via drill 0.41)
  Top 0.508: D10.C v70.17,9.05
  Bottom 0.508: JP8.5 v70.17,9.05 70.17,9.62 68.98,10.81 Q5.3
GPO3  (via drill 0.41)
  Top 0.508: D11.C v72.71,9.05
  Bottom 0.508: JP8.3 v72.71,9.05 72.71,10 71.9,10.81 Q6.3
GPO4  (via drill 0.41)
  Top 0.508: D12.C v75.25,9.05
  Bottom 0.508: Q7.3 v75.25,9.05 JP8.1
LCD_CS
  Bottom 0.508: HG1.1 74.3,49.37 71.44,46.51 68.58,46.51 67.58,45.52 IC2.30
LCD_D0
  Bottom 0.305: 85.73,43.02 88.27,43.02
  Bottom 0.508: IC2.35 73.62,40.75 75.88,43.02 85.73,43.02 | 88.27,43.02 HG1.6
LCD_D1
  Bottom 0.508: IC2.36 74.4,39.95 76.2,41.75 HG1.7
LCD_D2
  Bottom 0.305: 85.73,40.48 88.27,40.48
  Bottom 0.508: IC2.37 75.19,39.15 76.52,40.48 85.73,40.48 | 88.27,40.48 HG1.8
LCD_D3
  Bottom 0.508: IC2.38 75.98,38.35 76.84,39.21 HG1.9
LCD_D4
  Bottom 0.305: 85.73,37.94 88.27,37.94
  Bottom 0.508: IC2.39 76.77,37.55 77.15,37.94 85.73,37.94 | 88.27,37.94 HG1.10
LCD_D5
  Bottom 0.508: IC2.40 77.55,36.75 77.79,36.99 86.68,36.99 HG1.11 86.91,36.75
LCD_D6
  Bottom 0.305: 85.73,35.4 88.27,35.4
  Bottom 0.508: IC2.41 85.17,35.95 85.73,35.4 | 88.27,35.4 HG1.12
LCD_D7
  Bottom 0.508: IC2.42 84.7,35.15 85.73,34.13 HG1.13
LCD_D8
  Bottom 0.305: 85.73,32.86 88.27,32.86
  Bottom 0.508: IC2.51 67.58,27.19 68.58,26.19 70.8,26.19 72.07,27.46 75.88,27.46 83.82,31.91 85.41,32.86 85.73,32.86 | 88.27,32.86 HG1.14
LCD_D9  (via drill 0.41)
  Top 0.508: v84.77,30.96 84.14,31.59 v84.14,33.81
  Bottom 0.508: IC2.50 68.38,27.66 68.9,27.15 70.48,27.15 71.76,28.42 75.56,28.42 82.87,32.54 v84.14,33.81 | HG1.15 85.73,31.59 v84.77,30.96
LCD_D10  (via drill 0.41)
  Top 0.508: v83.19,30 82.23,30.96 v82.23,33.81
  Bottom 0.305: 88.27,30.32 86.04,30.32
  Bottom 0.406: 86.04,30.32 85.41,29.69
  Bottom 0.508: IC2.49 69.18,28.45 69.22,28.42 70.48,28.42 71.44,29.37 75.25,29.37 80.96,32.54 v82.23,33.81 | HG1.16 88.27,30.32 | 85.41,29.69 83.5,29.69 v83.19,30
LCD_D11  (via drill 0.41)
  Top 0.508: 81.28,29.37 v81.6,29.05 80.33,30.32 v80.33,33.81
  Bottom 0.508: IC2.48 74.96,30.35 79.06,32.54 v80.33,33.81 | HG1.17 86.36,29.05 86.04,28.73 81.92,28.73 v81.6,29.05
LCD_D12  (via drill 0.41)
  Top 0.508: v78.42,33.81 78.42,29.69 v80.01,28.1
  Bottom 0.305: 88.27,27.78 86.04,27.78
  Bottom 0.508: IC2.47 74.49,31.15 77.15,32.54 v78.42,33.81 | HG1.18 88.27,27.78 | 86.04,27.78 80.33,27.78 v80.01,28.1
LCD_D13  (via drill 0.41)
  Top 0.508: 78.11,27.46 v78.42,27.15 76.52,29.05 v76.52,33.81
  Bottom 0.508: IC2.46 74.02,31.95 75.25,32.54 v76.52,33.81 | HG1.19 79.06,26.51 v78.42,27.15
LCD_D14  (via drill 0.41)
  Top 0.508: 76.52,26.51 v76.84,26.19 74.61,28.42 v74.61,33.81
  Bottom 0.305: 88.27,25.24 86.04,25.24
  Bottom 0.508: IC2.45 73.55,32.75 v74.61,33.81 | HG1.20 88.27,25.24 | 86.04,25.24 77.79,25.24 v76.84,26.19
LCD_D15  (via drill 0.41)
  Top 0.508: v72.87,33.97 73.03,33.81 73.03,27.46 v75.25,25.24
  Bottom 0.508: IC2.44 72.45,33.55 v72.87,33.97 | HG1.21 76.52,23.97 v75.25,25.24
LCD_RD
  Bottom 0.305: 85.73,45.56 88.27,45.56
  Bottom 0.508: IC2.33 72.04,42.35 75.25,45.56 85.73,45.56 | 88.27,45.56 HG1.4
LCD_RS
  Bottom 0.305: 88.58,48.42 88.27,48.1 85.41,48.1
  Bottom 0.508: HG1.2 88.58,48.42 | 85.41,48.1 74.61,48.1 72.07,45.56 68.9,45.56 68.38,45.05 IC2.31
LCD_RST
  Bottom 0.508: IC2.34 72.83,41.55 75.56,44.29 HG1.5
LCD_WR
  Bottom 0.508: HG1.3 74.93,46.83 72.25,44.15 IC2.32
MISO  (via drill 0.41)
  Top 0.508: v81.92,16.35 78.42,19.84 60.96,19.84 54.29,26.51 54.29,28.1 55.56,29.37 55.56,35.08 51.44,39.21 v50.8,39.21
  Bottom 0.508: IC2.13 52.81,39.95 52.07,39.21 v50.8,39.21 | HG1.29 84.45,13.81 v81.92,16.35
MOSI  (via drill 0.41)
  Top 0.508: v81.92,14.45 81.6,14.45 77.15,18.89 60.33,18.89 53.34,25.88 53.34,29.37 54.61,30.64 54.61,34.45 51.91,37.15 v50.8,37.15
  Bottom 0.305: 88.27,12.54 85.73,12.54
  Bottom 0.508: HG1.30 88.27,12.54 | 85.73,12.54 83.82,12.54 v81.92,14.45 | IC2.12 53.6,39.15 51.59,37.15 v50.8,37.15
MUTE  (via drill 0.41)
  Top 0.508: IC4.1 26.67,18.89 28.89,21.11 41.59,21.11 | 41.59,21.11 R10.1 | v51.44,33.5 51.44,33.81 49.85,35.4 46.99,35.4 41.59,30 41.59,21.11
  Bottom 0.508: 51.44,33.81 v51.44,33.5 53.89,35.95 IC2.8
N$1  (via drill 0.41)
  Top 0.508: Q1.2 67.95,41.28 66.99,41.28 66.93,41.21 66.93,40.16 | C9.2 66.93,40.16 | v65.56,40.32 66.77,40.32 66.93,40.16
  Bottom 0.508: IC2.24 62.78,43.1 v65.56,40.32
N$2  (via drill 0.41)
  Top 0.508: Q1.1 59.69,41.28 60.64,41.28 60.7,41.21 60.7,40.48 | C8.2 60.7,40.48 | v62.07,40.32 60.86,40.32 60.7,40.48
  Bottom 0.508: IC2.23 61.98,40.55 v62.07,40.32
N$3
  Bottom 0.508: IC2.62 58.78,27.19 58.2,26.61 C7.2
N$4
  Bottom 0.508: R2.2 51.51,48.66 50.8,49.37 JP4.MISO
N$5
  Top 0.508: C16.+ 23.81,17.94 24.13,17.62 IC4.3
N$6
  Top 0.508: MODULE2.10 24.26,39.34 25.4,40.48 29.21,40.48 32.02,43.29 L1.2
  Top 0.813: C11.+ 19.37,36.99 | 19.37,36.99 20.32,36.99 21.59,38.26 MODULE2.10 | C12.1 16.83,35.72 18.1,36.99 19.37,36.99
N$7
  Top 0.508: C17.+ 24.13,21.11 25.4,19.84 IC4.2
N$8  (via drill 0.41)
  Top 0.508: MODULE2.5 32.26,27.59 30.48,29.37 v20.95,29.37
  Bottom 0.508: v20.95,29.37 13.34,29.37 11.11,27.15 JP7.1
N$9
  Top 0.508: C13.+ 21.91,24.61 23.18,23.34 25.72,23.34 26.26,23.88 MODULE2.2
N$10
  Top 0.508: R19.2 17.46,24.52 C13.-
N$11
  Top 0.61: IC4.6 24.13,11.91
  Top 0.813: 24.13,11.91 24.13,12.54 24.77,13.18 28.57,13.18 29.53,14.13 31.43,14.13 | 31.43,14.13 C19.+ | C21.2 36.1,13.59 35.56,14.13 35.24,14.13 | 35.24,14.13 31.43,14.13 | L2.2 35.24,14.13
N$12
  Top 0.508: C15.+ 13.65,15.08 13.65,17.3 13.02,17.94 R21.2 R20.1
N$13
  Top 0.508: 20.64,15.08 C15.- 16.83,15.17 16.83,17.3 17.46,17.94 R19.1 | 20.64,15.08 22.8,15.08 IC4.4 | R22.2 20.64,15.08
N$14
  Top 0.61: IC4.8 26.67,8.41 26.04,7.78 JP9.1
N$15
  Top 0.508: R22.1 20.64,10 21.59,9.05 22.86,9.05
  Top 0.61: IC4.5 22.86,9.05 22.86,8.41 23.5,7.78 JP9.2
N$16
  Bottom 0.508: SJ2.2 6.03,47.78 7.3,49.05 JP3.1
N$17
  Top 0.508: Q2.3 14.46,48.59 14.92,49.05 JP3.4
N$18  (via drill 0.41)
  Top 0.508: v55.56,46.04 55.56,47.9 D4.C
  Bottom 0.508: R5.2 47.62,38.26 48.26,38.89 48.26,41.43 51.44,44.61 51.44,45.38 R2.1 51.51,45.64 51.75,45.88 55.4,45.88 v55.56,46.04
N$19
  Top 0.508: Q2.1 16.66,44.14 17.14,43.66 21.91,43.66 33.97,55.72 67.63,55.72 | Q3.3 69.7,53.65 67.63,55.72 | 67.63,55.72 R4.1
N$20
  Top 0.508: MODULE1.1 11.43,36.57 C10.1
  Bottom 0.508: SJ4.2 6.03,41.75 8.57,39.21 MODULE1.1
N$23
  Top 0.508: SJ3.2 D3.A
  Top 0.813: D3.A JP4.+5V
N$25
  Bottom 0.508: JP4.MOSI 48.26,50.01 49.21,49.05 D5.C
N$26
  Bottom 0.508: D6.C 53.66,48.42 53.34,48.74 JP4.SCK
PDI(MOSI)/RX
  Bottom 0.508: 47.31,41.12 47.31,42.07 49.21,43.97 D5.A | 47.31,41.12 47.31,39.85 45.72,38.26 45.72,33.81 48.38,31.15 IC2.2 | R9.2 47.31,41.12
PDO(MISO)/TX
  Bottom 0.508: IC2.3 48.85,31.95 47.62,33.18 R5.1
PHOTO
  Bottom 0.508: 61.28,10.64 61.28,20.16 61.18,20.26 IC2.59 | 61.28,10.64 61.28,9.68 63.18,7.78 JP2.1 | R3.2 61.28,10.64
RESET
  Bottom 0.508: IC2.20 59.58,45.99 55.88,49.69 JP4.RST R8.2
SCK  (via drill 0.41)
  Top 0.508: v49.53,33.5 49.53,32.23 51.44,30.32 51.44,24.61 55.88,20.16 | 55.88,20.16 59.05,16.99 75.25,16.99 81.28,10.95 v81.28,7.46 | R7.2 55.25,19.53 55.88,20.16
  Bottom 0.508: HG1.34 87.95,7.14 82.55,7.14 82.23,7.46 v81.28,7.46 | 49.53,35.08 49.21,35.4 49.21,41.12 52.33,44.23 D6.A | 49.53,35.08 v49.53,33.5 | 49.53,35.08 51.12,35.08 54.39,38.35 IC2.11
SCL  (via drill 0.41)
  Top 0.508: v21.91,35.72 29.53,35.72 30.26,36.45 MODULE2.7 30.26,39.94 31.75,41.43 46.36,41.43 49.53,44.61 56.2,44.61 v62.23,50.64 65.09,50.64 67.16,48.57 73.18,48.57 74.45,49.85 IC3.16
  Bottom 0.508: IC2.25 63.58,48.97 62.23,50.32 v62.23,50.64 62.55,50.96 62.55,52.86 R17.2 | v21.91,35.72 20,35.72 MODULE1.3
SD_CS  (via drill 0.41)
  Top 0.508: v73.66,24.29 71.44,26.51 71.44,30 v67.95,33.5
  Bottom 0.305: 88.27,22.7 86.04,22.7
  Bottom 0.508: HG1.22 88.27,22.7 | 86.04,22.7 81.92,22.7 | 81.92,22.7 75.25,22.7 v73.66,24.29 | 82.23,22.07 R24.2 81.92,22.7 | IC2.29 66.78,42.28 67.31,41.75 67.31,34.77 67.95,34.13 v67.95,33.5
SDA  (via drill 0.41)
  Top 0.508: IC3.15 76.2,48.1 75.56,47.47 66.04,47.47 v64.77,48.74 61.91,48.74 56.83,43.66 50.17,43.66 46.99,40.48 32.7,40.48 32.26,40.04 MODULE2.6 32.26,35.91 30.16,33.81 v21.91,33.81
  Bottom 0.508: IC2.26 64.38,48.75 | 64.38,48.75 64.38,54.52 63.5,55.4 R18.2 | MODULE1.4 20.64,39.21 23.5,36.35 23.5,35.08 22.22,33.81 v21.91,33.81 | 64.38,48.75 v64.77,48.74
SENSOR_RX  (via drill 0.41)
  Top 0.508: JP3.3 12.38,47.15 | 12.38,47.15 12.38,45.56 15.24,42.7 22.54,42.7 33.66,53.82 66.36,53.82 v66.67,53.5 | D2.C 12.38,47.15
  Bottom 0.508: R1.2 JP3.3 | v66.67,53.5 66.67,47.78 65.18,46.29 IC2.27
SENSOR_TX  (via drill 0.41)
  Top 0.508: Q3.1 68.75,51.45 v68.58,51.28
  Bottom 0.508: IC2.28 65.98,45.5 68.58,48.1 v68.58,51.28 R6.1
SOUND  (via drill 0.41)
  Top 0.508: v53.66,42.07 53.02,42.39 50.8,42.39 39.37,30.96 v39.37,27.78 | v15.24,24.61 R20.2
  Bottom 0.508: IC2.16 54.01,42.35 v53.66,42.07 | v39.37,27.78 25.08,27.78 22.86,25.56 16.19,25.56 v15.24,24.61
SUPPLY  (via drill 0.41)
  Top 0.406: U1.VBUS1 25.75,53.47 26.04,53.18
  Top 0.813: 26.04,53.18 26.04,52.23 JP1.1 21.59,46.2 20.64,45.24 v18.1,45.24
  Bottom 0.813: v18.1,45.24 17.46,45.24 15.46,47.24 D1.A SJ1.2
T_CS
  Bottom 0.508: 69.22,20.16 65.18,24.19 IC2.54 | 69.22,20.16 71.12,18.26 76.2,18.26 78.42,16.03 78.42,11.91 81.6,8.73 HG1.33 | R23.2 69.22,20.16
T_PEN  (via drill 0.41)
  Top 0.508: v53.34,33.5 53.34,31.27 52.39,30.32 52.39,25.24 59.69,17.94 76.2,17.94 81.6,12.54 v81.92,12.54
  Bottom 0.508: IC2.6 54.2,34.35 v53.34,33.5 | v81.92,12.54 83.19,11.27 HG1.31
UART_SPD
  Bottom 0.305: 54.61,51.91 54.61,49.37
  Bottom 0.508: SJ5.2 55.56,53.5 54.61,52.55 54.61,51.91 | 54.61,49.37 57.18,46.8 IC2.17
VBAT  (via drill 0.41)
  Top 0.508: IC3.14 77.47,52.23 77.06,52.64 C14.2 75.88,53.5 72.07,49.69 67.95,49.69 65.09,52.55 47.31,52.55 45.72,50.96 v45.72,45.24
  Bottom 0.508: v45.72,45.24 GB1.GB+
VCC  (via drill 0.41)
  Top 0.508: C6.2 57.79,31.91 | R10.2 49.85,21.11 | R4.2 v73.66,55.72 | R7.1 49.85,19.53
  Top 0.813: v57.47,31.91 57.79,31.91 v64.77,31.91 65.72,31.91 66.67,30.96 C5.2 | IC3.2 76.2,37.94 | 76.2,37.94 C20.2 | 76.2,37.94 70.8,37.94 v68.9,36.04 | v49.85,29.37 49.85,21.11 49.85,19.53 49.85,12.22 | 49.85,12.22 48.58,12.22 JP5.1 | 49.85,12.22 56.52,12.22 | 56.52,12.22 76.52,12.22 77.47,11.27 77.47,5.87 79.38,3.97 82.87,3.97 85.09,6.19 v85.09,10 | v39.69,46.51 38.1,46.51 37.42,47.19 L1.1 | JP6.1 56.52,12.22
  Bottom 0.305: 88.27,10 85.73,10
  Bottom 0.508: IC2.64 57.18,29.35 | 57.18,29.35 57.18,30.12 57.23,30.16 | IC2.52 66.78,30.85 66.67,30.96 | 59.69,42.7 60.38,43.4 IC2.21 60.38,47.09 59.91,47.56 | 60.23,50.76 R8.1 | 69.22,34.45 69.37,34.45 69.37,32.54 69.22,32.54 | SJ4.3 SJ2.3 | 80.01,20.16 R23.1 | 57.18,29.35 57.17,29.35 57.15,29.37 56.83,29.37 | 43.82,10.1 R11.1 | 56.52,10.1 R12.1 R3.1 | HG1.32 88.27,10 | 85.73,10 v85.09,10 | R9.1 44.45,40.8 | SJ5.3 R18.1 | v73.66,55.72 70.17,55.72 69.85,55.4 68.8,55.4 R6.2
  Bottom 0.813: HG1.24 HG1.25 84.77,18.89 83.5,20.16 81.92,20.16 | 57.23,30.16 57.23,31.67 v57.47,31.91 59.05,33.5 59.05,42.07 59.69,42.7 | v64.77,31.91 65.72,31.91 66.67,30.96 68.26,30.96 69.22,31.91 69.22,32.54 | 59.91,47.56 C4.2 59.91,48.96 60.11,49.15 R8.1 | 60.23,50.76 R17.1 R18.1 60.23,56.26 60.96,56.99 67.95,56.99 68.58,56.36 R6.2 | v68.9,36.04 69.22,35.72 69.22,34.45 | v39.69,46.51 C3.+ | 12.38,54.45 18.73,54.45 22.54,50.64 24.77,50.64 28.89,46.51 32.73,46.51 | 12.38,54.45 7.62,54.45 4.45,51.28 4.45,47.78 4.51,47.72 SJ2.3 | R1.1 12.38,54.45 | R24.1 81.92,20.16 | 81.92,20.16 80.01,20.16 80.01,18.26 | 56.83,29.37 v49.85,29.37 48.58,29.37 44.45,33.5 44.45,40.8 44.45,43.97 41.91,46.51 v39.69,46.51 | JP5.1 43.82,10.1 | JP6.1 56.52,10.1 | v39.69,46.51 32.73,46.51 | 32.73,46.51 IC1.4 | v85.09,10 82.23,10 80.01,12.22 80.01,18.26 | C18.2 80.01,18.26
  pour Bottom (isolate 0.61): 42.23,50.32 42.23,41.43 19.37,41.43 19.37,47.78 12.38,54.77 12.07,54.77 12.07,57.94 52.39,57.94 52.39,50.32
  pour Bottom (no thermals): 29.85,44.29 35.56,44.29 35.56,49.05 29.85,49.05
WIRE1
  Bottom 0.508: JP5.3 38.73,9.89 | 38.73,9.89 D7.C R11.2 | 38.73,9.89 38.73,12.22 40.64,14.13 51.12,14.13 59.58,22.59 IC2.61
WIRE2
  Bottom 0.508: JP6.3 51.44,9.89 | 51.44,9.89 D8.C R12.2 | 51.44,9.89 51.44,12.22 60.38,21.17 IC2.60

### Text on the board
tPlace: Rx | Tx | VCC | Gnd | VCC | Gnd | MO/Rx | MI/Tx | SCK | Rst | uUSB | | | 1 | 2 | 3 | 4 | Open | DQ | DQ | drain | Gnd | Vdd | Gnd | Vdd | Gnd
bPlace: 9600 | UART | 1200 | UART pwr | 3v3 | 5v0 | + - | TOUCH CLOCK v.2 | (c) GoldenAndy 2019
